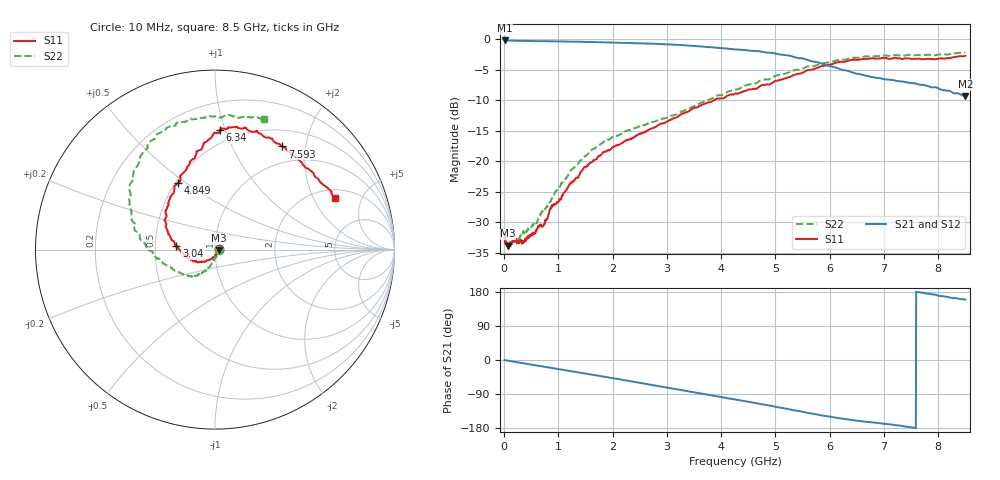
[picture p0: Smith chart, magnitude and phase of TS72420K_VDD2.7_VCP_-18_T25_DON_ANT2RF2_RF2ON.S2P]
!Agilent Technologies,E5071C,MY46417908,A.11.23
!Date: Thu Oct 03 16:41:00 2019
!Data & Calibration Information:
!Freq	S11:SOLT2(ON)	S21:SOLT2(ON)	S12:SOLT2(ON)	S22:SOLT2(ON)
!PortZ  Port1:50+j0  Port2:50+j0
!Above PortZ is port z conversion or system Z0 setting when saving the data.
!When reading, reference impedance value at option line is always used.
# Hz S dB R 50
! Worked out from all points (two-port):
!   1601 points, 10 MHz to 8.5 GHz, reference 50 ohm
!   highest |S21| = -0.25 dB at 10 MHz (marker M1); lowest = -9.4 dB at 8.5 GHz (marker M2)
!   |S21| within 3 dB of the highest: start of sweep to 5.533 GHz
!   lowest |S11| = -33.8 dB at 68.37 MHz (marker M3), VSWR 1.04, Z = 52.1 - j0.359 ohm
!   |S11| at or under -10 dB: start of sweep to 3.879 GHz
!   |S22| runs from -33.9 to -2.2 dB; largest |S21 - S12| = 0.0055
!   S11 on the Smith chart (normalised r, x): 10 MHz: 1.05, +0.01; 3.04 GHz: 0.65, +0.03; 4.849 GHz: 0.51, +0.46; 6.34 GHz: 0.40, +0.96; 7.593 GHz: 0.73, +1.60; 8.5 GHz: 2.43, +2.99
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1e7  -32.50 9.8  -0.25 -0.3  -0.25 -0.3  -33.23 -10.7
6.836875e7  -33.78 -9.7  -0.28 -1.7  -0.28 -1.7  -33.48 -14.8
1.3735e8  -33.48 -12.3  -0.29 -3.4  -0.30 -3.4  -33.60 -20.6
3.602125e8  -33.32 -39.4  -0.32 -8.8  -0.33 -8.7  -31.38 -47.8
5.83075e8  -31.42 -73.0  -0.35 -14.0  -0.36 -14.0  -30.00 -69.7
7.3165e8  -30.46 -85.3  -0.37 -17.5  -0.37 -17.5  -28.00 -76.2
8.80225e8  -27.14 -93.8  -0.39 -21.0  -0.39 -20.9  -26.18 -92.6
1.023494e9  -26.19 -106.7  -0.40 -24.4  -0.40 -24.3  -24.20 -96.1
1.230438e9  -23.55 -119.7  -0.44 -29.3  -0.43 -29.3  -21.44 -104.2
1.426769e9  -21.65 -129.0  -0.48 -34.0  -0.47 -34.0  -19.77 -109.1
2.010456e9  -17.62 -149.9  -0.58 -48.0  -0.58 -47.9  -15.95 -120.0
2.843538e9  -14.08 -179.7  -0.82 -68.6  -0.82 -68.6  -13.26 -138.6
3.039869e9  -13.30 174.7  -0.90 -73.5  -0.90 -73.4  -12.74 -145.5
3.591719e9  -10.97 159.1  -1.20 -87.5  -1.20 -87.5  -10.61 -164.4
4.255e9  -8.94 138.3  -1.71 -104.1  -1.72 -103.9  -8.29 176.6
4.8493e9  -7.44 119.3  -2.23 -119.0  -2.24 -119.0  -6.63 162.1
5.284412e9  -6.15 107.4  -2.78 -131.2  -2.79 -131.2  -5.33 151.6
5.671769e9  -5.01 98.6  -3.67 -141.3  -3.65 -141.2  -4.46 139.6
6.340356e9  -3.54 87.6  -5.25 -156.8  -5.27 -156.7  -3.23 123.0
7.088538e9  -3.26 73.6  -6.65 -169.6  -6.69 -169.5  -2.77 108.4
7.592631e9  -3.26 56.8  -7.31 180.0  -7.24 179.8  -2.65 97.4
8.5e9  -2.75 23.4  -9.38 159.4  -9.43 159.3  -2.18 69.6
